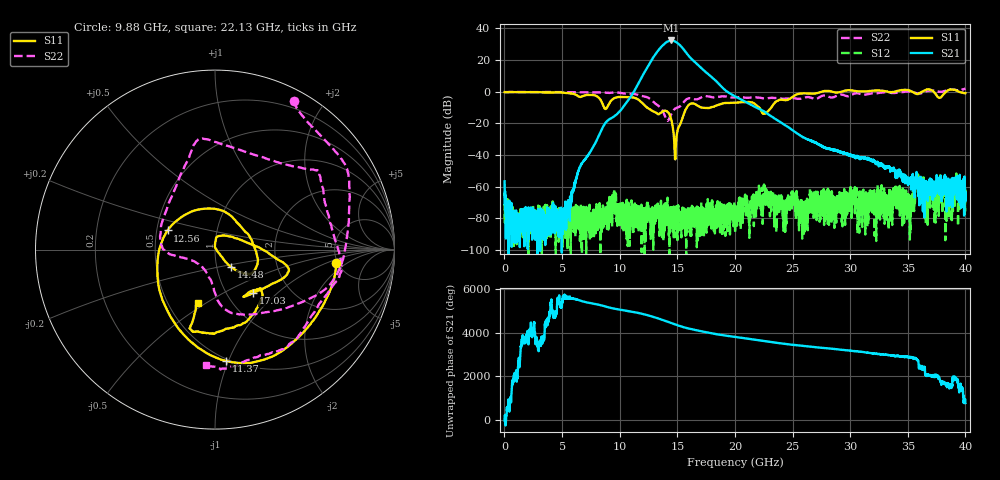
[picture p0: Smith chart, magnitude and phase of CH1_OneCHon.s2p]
!Keysight Technologies,N5245B,MY57181321,A.14.80.03
!Date: Thursday, August 24, 2023 18:01:01
!Correction: S11(C  2-Port  )
!S21(C  2-Port  )
!S12(C  2-Port  )
!S22(C  2-Port  )
!S2P File: Measurements: S11, S21, S12, S22:
# Hz S  RI  R 50
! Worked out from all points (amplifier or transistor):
!   4000 points, 10 MHz to 40 GHz, reference 50 ohm
!   highest |S21| = 32.4 dB at 14.44 GHz (marker M1)
!   |S21| within 3 dB of that: 13.75 GHz to 15.23 GHz (1.483 GHz wide, 10.2 % of centre)
!   unconditionally stable (mu >= 1): start of sweep to 27.53 GHz; 28.44 GHz to 29.22 GHz; 35.41 GHz to 36.24 GHz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
!   at 6.67 GHz: K = 39338.83, MAG = -31.8 dB, |S12| = -80.1 dB
!   at 20.01 GHz: K = 9267.38, MAG = 0.5 dB, |S12| = -89.3 dB
!   at 40 GHz: K = -370446.88, MSG = 0.0 dB, |S12| = -68.7 dB
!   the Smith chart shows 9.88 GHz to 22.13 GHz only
!   S11 on the Smith chart (normalised r, x): 9.88 GHz: 4.83, -1.38; 11.37 GHz: 0.48, -0.98; 12.56 GHz: 0.57, +0.13; 14.48 GHz: 1.17, -0.23; 17.03 GHz: 1.32, -0.71; 22.13 GHz: 0.70, -0.46
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1e7  -0.9696 0.0443  0.0011 -0.00098  0.000408 0.000296  -0.9706 0.0216
6.68e9  0.4064 0.5647  0.00334 0.00401  0.000159 -8.13e-05  -0.3668 0.8875
9.88e9  0.6749 -0.0768  0.1911 0.0963  -4.81e-05 6.52e-05  0.4391 0.8287
1.137e10  0.064 -0.6207  -0.4421 -1.148  -1.88e-05 -7.35e-05  0.7475 0.3681
1.256e10  -0.2639 0.107  -0.8959 7.455  -8.54e-05 3.54e-05  0.5624 -0.2552
1.296e10  -0.0499 0.2282  10.71 7.274  -8.72e-05 -4.38e-09  0.31 -0.3453
1.334e10  0.1378 0.136  17.35 -10.15  -0.000146 9.91e-05  0.0895 -0.3521
1.385e10  0.2367 -0.082  -17.04 -26.89  2.23e-05 2.24e-05  -0.015 -0.195
1.416e10  0.1836 -0.136  -38.45 1.017  0.000188 0.000187  -0.0778 -0.092
1.444e10  0.1005 -0.103  -23.32 34.44  -0.000109 0.000179  -0.1784 -0.0453
1.448e10  0.0882 -0.0958  -18.42 37.11  3.65e-05 -0.000102  -0.1938 -0.0416
1.472e10  0.0224 -0.0201  13.5 37.49  0.000217 4.68e-05  -0.271 -0.0133
1.503e10  0.00542 0.062  33.21 7.908  -2.39e-05 3.69e-05  -0.3032 0.0874
1.529e10  0.0655 0.0769  23.78 -14.55  -3.18e-05 1.24e-05  -0.2622 0.2455
1.554e10  0.1822 0.0377  6.819 -20.88  4.26e-05 -0.000102  -0.1887 0.4226
1.609e10  0.3988 -0.0878  -10.14 -6.921  -0.000119 7.01e-05  -0.0785 0.6164
1.703e10  0.2109 -0.2421  -1.597 5.618  6.39e-05 -3.34e-05  0.4577 0.4608
2.001e10  0.0655 -0.4412  -0.6516 -0.282  3.21e-05 1.24e-05  0.499 -0.4308
2.213e10  -0.0955 -0.2951  0.2084 0.1947  0.00028 0.000653  -0.049 -0.644
2.667e10  -0.5154 -0.7098  -0.00873 0.0262  0.000263 0.000113  -0.3916 0.4962
3.334e10  -0.6799 0.6972  -0.00015 0.00434  -3.87e-05 1.91e-05  0.9069 -0.2505
4e10  0.8635 0.2676  0.000262 0.000265  1.23e-08 0.000369  0.1399 -1.241
